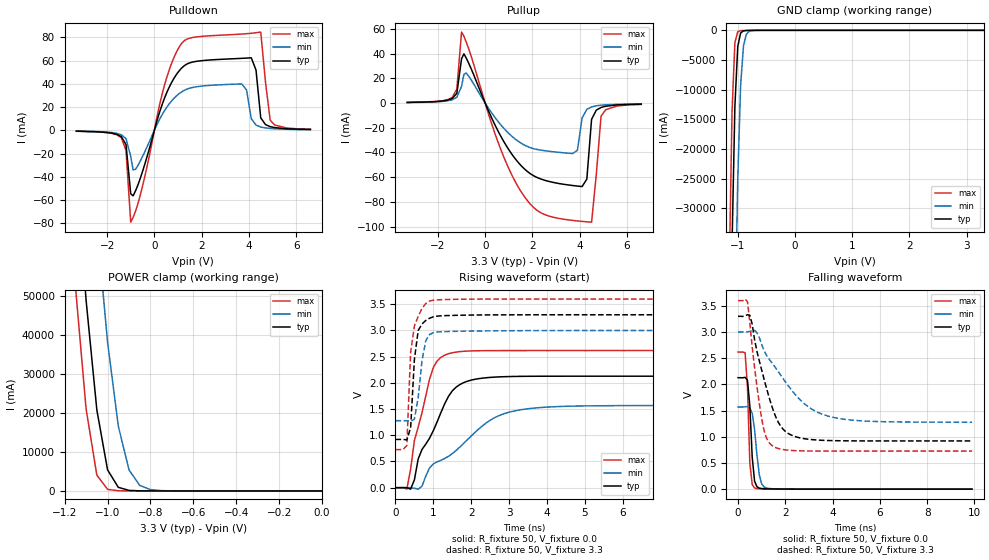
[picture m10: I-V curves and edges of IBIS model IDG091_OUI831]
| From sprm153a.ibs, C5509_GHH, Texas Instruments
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| Pin_model   IDG091_OUI831
[Model]   IDG091_OUI831
 Model_type   I/O
 Polarity   Non-Inverting
 Enable   Active-Low
 Vinl  =  1.08
 Vinh  =  2.1
 Vmeas =  1.5
|Variable   typ   min   max
 C_comp   2.046pF   2.03pF   2.12pF
[Temperature Range]   25   125   -40
[Voltage Range]   3.3   3   3.6
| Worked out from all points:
|   slope of the pulldown table from 0 to 0.495 V, typ, clamps not added: 16 ohm
|   slope of the pullup table from 0 to 0.495 V, typ, clamps not added: 23.8 ohm
|   GND clamp passes 1 mA (typ) near -0.59 V on its own axis
|   POWER clamp passes 1 mA (typ) near -0.70 V on its own axis
|   rising waveform, R_fixture 50, V_fixture 0.0: 20-80 % time 802ps typ, 1.58ns min, 480ps max; typ from 0 V to 2.13 V
|   rising waveform, R_fixture 50, V_fixture 3.3: 20-80 % time 148ps typ, 184ps min, 159ps max; typ from 0.921 V to 3.3 V
|   falling waveform, R_fixture 50, V_fixture 0.0: 20-80 % time 164ps typ, 228ps min, 121ps max; typ from 2.13 V to 0 V
|   falling waveform, R_fixture 50, V_fixture 3.3: 20-80 % time 868ps typ, 1.74ns min, 488ps max; typ from 3.3 V to 0.921 V
[GND Clamp]
|Voltage   I(typ)   I(min)   I(max)
-3.3V     -2.131kA   -2.172kA   -2.112kA
-1.15V    -69.25A    -121A      -41.3A
-1.1V     -36.04A    -83.7A     -13.64A
-1.05V    -12.77A    -50.83A    -2.067A
-1V       -2.726A    -25.08A    -235.7mA
-950mV    -452.7mA   -9.272A    -58.81mA
-900mV    -87.44mA   -2.634A    -35.32mA
-850mV    -28.97mA   -661.7mA   -25.37mA
-800mV    -15.75mA   -165.5mA   -17.41mA
-600mV    -1.159mA   -2.524mA   -779.4uA
3.3V      218.1pA    2.598nA    184.3pA
[POWER Clamp]
|Voltage   I(typ)   I(min)   I(max)
-3.3V     2.152kA    2.199kA    2.128kA
-1.15V    84.65A     142.8A     52.53A
-1.1V     48.8A      103.8A     20.98A
-1.05V    20.76A     68.2A      4.051A
-1V       5.397A     38.14A     408.9mA
-950mV    921mA      16.63A     39.31mA
-900mV    138.5mA    5.377A     6.91mA
-850mV    22mA       1.408A     3.323mA
-800mV    4.66mA     339.8mA    2.313mA
-750mV    1.713mA    80.91mA    1.624mA
0V        0A         0A         0A
[Pulldown]
|Voltage   I(typ)   I(min)   I(max)
-3.3V     -700uA     -600uA     -800uA
-1.4V     -5.37mA    -3.81mA    -6.26mA
-1.2V     -12.25mA   -7.11mA    -17.31mA
-1V       -54.58mA   -22.44mA   -78.99mA
-800mV    -52.16mA   -33.54mA   -69.68mA
400mV     26.07mA    15.89mA    36.64mA
1.1V      52.31mA    32.25mA    73.11mA
3.7V      61.86mA    39.87mA    82.75mA
4.1V      62.32mA    9.97mA     83.41mA
4.5V      10.72mA    2.83mA     84.43mA
4.9V      3.13mA     1.59mA     8.65mA
6.6V      700uA      600uA      1mA
[Pullup]
|Voltage   I(typ)   I(min)   I(max)
-3.3V     500uA      500uA      600uA
-1.4V     3.68mA     2.67mA     4.45mA
-1.2V     7.89mA     4.73mA     11.41mA
-1V       35.94mA    13.64mA    57.52mA
850mV     -33.18mA   -21.68mA   -46.54mA
2.15V     -59.85mA   -37.37mA   -86.19mA
3.7V      -66.75mA   -40.84mA   -95.02mA
4.1V      -67.58mA   -12.01mA   -95.82mA
4.3V      -61.52mA   -5.05mA    -96.15mA
4.5V      -13.12mA   -3.07mA    -96.45mA
4.9V      -3.53mA    -1.69mA    -10.6mA
6.6V      -800uA     -600uA     -1.1mA
[Ramp]
|Variable   typ   min   max
 dV/dt_r   1.29V/0.810ns   0.94V/1.580ns   1.59V/0.490ns
 dV/dt_f   1.43V/0.870ns   1.03V/1.740ns   1.73V/0.490ns
 R_load =  50
[Rising Waveform]
 R_fixture =   50
 V_fixture =   0.0
 V_fixture_min =  0.0
 V_fixture_max =  0.0
|Time   V(typ)   V(min)   V(max)
0s        15.59nV    2.851uV    10.25nV
300ps     -531.8uV   1.305mV    -27mV
500ps     150.6mV    -11.48mV   901.1mV
600ps     547.8mV    -27.49mV   1.159V
900ps     944.5mV    376.9mV    2.07V
1.1ns     1.257V     492.8mV    2.419V
1.4ns     1.743V     599.1mV    2.557V
2ns       2.053V     986.1mV    2.61V
3.3ns     2.125V     1.486V     2.617V
9.9ns     2.128V     1.569V     2.617V
[Rising Waveform]
 R_fixture =   50
 V_fixture =   3.3
 V_fixture_min =  3
 V_fixture_max =  3.6
|Time   V(typ)   V(min)   V(max)
0s        920.7mV    1.278V     727mV
300ps     910.9mV    1.278V     806.4mV
400ps     1.142V     1.262V     2.587V
500ps     2.451V     1.311V     3.09V
600ps     3.001V     1.717V     3.268V
700ps     3.124V     2.425V     3.421V
800ps     3.191V     2.806V     3.516V
900ps     3.235V     2.922V     3.562V
2.1ns     3.296V     2.99V      3.599V
9.9ns     3.3V       3V         3.6V
[Falling Waveform]
 R_fixture =   50
 V_fixture =   0.0
 V_fixture_min =  0.0
 V_fixture_max =  0.0
|Time   V(typ)   V(min)   V(max)
0s        2.128V     1.569V     2.617V
300ps     2.135V     1.573V     2.606V
400ps     2.078V     1.577V     1.943V
500ps     1.587V     1.55V      498.1mV
600ps     611.7mV    1.448V     89.63mV
700ps     152.9mV    1.139V     22.11mV
900ps     20.17mV    275.7mV    7.552mV
1ns       11.14mV    101.5mV    6.05mV
1.2ns     6.477mV    21.65mV    4.114mV
9.9ns     -33.95nV   2.56uV     22.12nV
[Falling Waveform]
 R_fixture =   50
 V_fixture =   3.3
 V_fixture_min =  3
 V_fixture_max =  3.6
|Time   V(typ)   V(min)   V(max)
0s        3.3V       3V         3.6V
400ps     3.331V     3.003V     3.58V
600ps     3.148V     3.027V     2.711V
1ns       2.275V     2.764V     1.347V
1.2ns     1.935V     2.561V     980.4mV
1.5ns     1.492V     2.371V     814.1mV
2.2ns     1.044V     1.929V     741.3mV
3ns       951.7mV    1.564V     728.9mV
3.8ns     929mV      1.396V     727mV
9.9ns     920.7mV    1.278V     727mV
